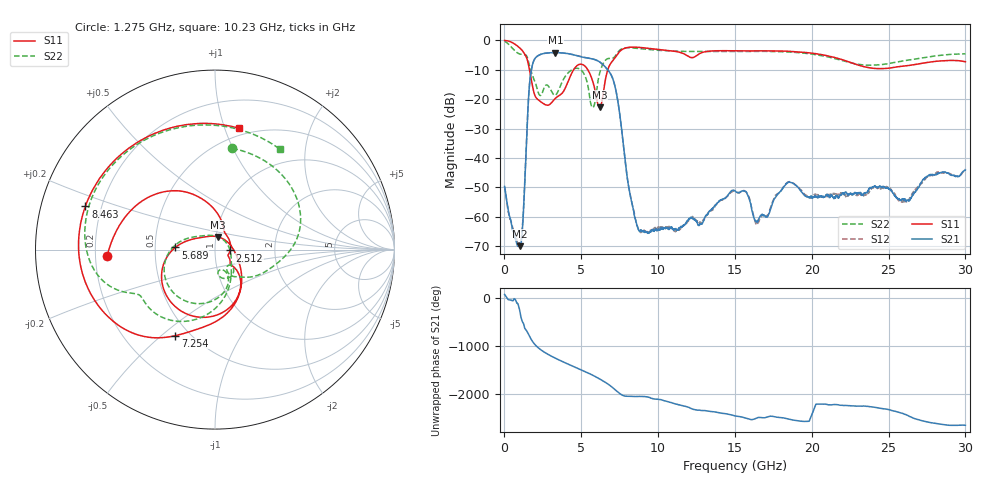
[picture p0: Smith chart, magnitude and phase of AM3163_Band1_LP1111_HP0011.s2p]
!Agilent Technologies,E8364B,MY43040894,A.07.50.67
!Agilent E8364B: A.07.50.67
!Date: Thursday, August 20, 2020 11:57:22
!Correction: S11(Full 2 Port(1,2))
!S21(Full 2 Port(1,2))
!S12(Full 2 Port(1,2))
!S22(Full 2 Port(1,2))
!S2P File: Measurements: S11, S21, S12, S22:
# Hz S  dB  R 50
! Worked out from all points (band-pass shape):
!   3201 points, 10 MHz to 30 GHz, reference 50 ohm
!   highest |S21| = -4.23 dB at 3.318 GHz (marker M1); lowest = -69.9 dB at 1.022 GHz (marker M2)
!   |S21| within 3 dB of the highest: 1.887 GHz to 6.151 GHz (4.264 GHz wide, 106 % of centre)
!   lowest |S11| = -22.7 dB at 6.186 GHz (marker M3), VSWR 1.16, Z = 51.3 + j7.29 ohm
!   |S11| at or under -10 dB: 1.626 GHz to 4.506 GHz (2.88 GHz wide, 93.9 % of centre); 5.418 GHz to 6.728 GHz (1.31 GHz wide, 21.6 % of centre)
!   |S22| runs from -22.9 to -0.4 dB; largest |S21 - S12| = 0.0044
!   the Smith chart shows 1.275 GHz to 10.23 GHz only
!   S11 on the Smith chart (normalised r, x): 1.275 GHz: 0.25, -0.03; 2.512 GHz: 1.18, -0.01; 5.689 GHz: 0.64, +0.02; 7.254 GHz: 0.42, -0.56; 8.463 GHz: 0.14, +0.16; 10.23 GHz: 0.44, +1.12
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1e7  -0.10 -8.6  -49.68 70.2  -49.74 32.5  -0.39 -15.2
4.411062e8  -0.65 -56.4  -62.02 -48.7  -61.85 -47.2  -2.31 -94.7
1.022162e9  -2.78 -134.9  -69.93 47.8  -69.14 57.4  -4.73 142.2
1.275203e9  -4.41 -176.6  -53.90 138.8  -53.49 98.5  -4.85 80.3
1.725053e9  -12.77 92.1  -10.92 -137.2  -10.92 -137.3  -10.34 -24.2
2.081184e9  -19.65 53.6  -5.67 74.1  -5.68 74.1  -15.62 -58.8
2.512291e9  -21.46 -3.2  -4.57 -34.9  -4.57 -34.9  -17.14 -44.3
3.318272e9  -19.72 -35.8  -4.23 -178.6  -4.24 -178.6  -18.64 -72.8
3.983675e9  -15.98 -43.1  -4.45 81.4  -4.47 81.4  -12.10 -79.9
5.014581e9  -8.17 -119.7  -5.67 -64.8  -5.65 -64.6  -10.25 -157.2
5.689356e9  -13.10 176.9  -6.33 -164.2  -6.30 -164.2  -22.66 77.6
6.186066e9  -22.75 75.9  -7.35 110.9  -7.39 110.8  -11.40 -78.5
7.254459e9  -5.55 -114.7  -17.08 -130.0  -17.07 -129.3  -5.09 -154.8
8.463431e9  -2.37 161.6  -59.72 103.6  -59.12 102.8  -2.69 131.9
1.000979e10  -3.12 88.2  -64.47 43.6  -63.48 41.8  -3.45 65.5
1.023472e10  -3.24 78.6  -63.89 33.9  -63.49 25.2  -3.53 56.9
1.5005e10  -3.59 -72.0  -51.18 59.2  -51.48 60.7  -3.79 -92.6
1.642952e10  -3.62 -106.4  -61.67 13.3  -62.56 15.0  -3.79 -127.4
2.000958e10  -4.40 162.5  -53.43 86.2  -53.22 -53.4  -4.71 135.4
2.274617e10  -7.98 59.6  -52.13 -95.3  -52.07 -94.0  -7.94 20.1
2.500479e10  -9.51 -63.0  -50.34 -170.1  -50.14 -171.9  -7.96 -93.2
3e10  -7.30 104.0  -44.10 -137.5  -43.71 -135.0  -4.65 100.3
